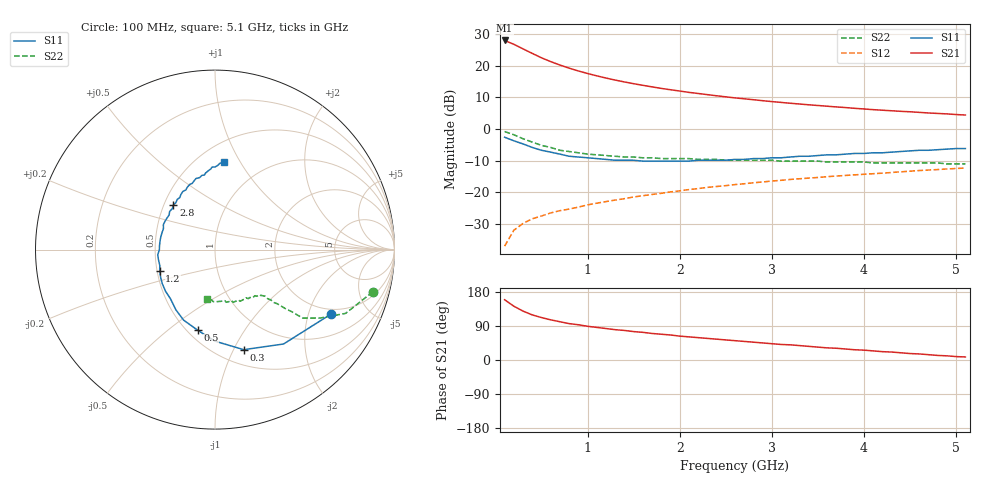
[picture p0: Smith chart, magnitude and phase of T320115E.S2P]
!AT-32011
!S PARAMETERS at Vce=5  V  Ic=10mA.  LAST UPDATED 01-05-95
# ghz s ma r 50
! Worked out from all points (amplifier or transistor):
!   51 points, 100 MHz to 5.1 GHz, reference 50 ohm
!   highest |S21| = 28.0 dB at 100 MHz (marker M1)
!   |S21| within 3 dB of that: start of sweep to 323.5 MHz
!   unconditionally stable (mu >= 1): 1.505 GHz to 4.873 GHz
!   at 900 MHz: K = 0.86, MSG = 21.5 dB, |S12| = -24.7 dB
!   at 2.6 GHz: K = 1.08, MAG = 11.9 dB, |S12| = -17.6 dB
!   at 5.1 GHz: K = 1.00, MSG = 8.4 dB, |S12| = -12.4 dB
!   S11 on the Smith chart (normalised r, x): 100 MHz: 1.79, -2.83; 300 MHz: 0.65, -1.10; 500 MHz: 0.56, -0.64; 1.2 GHz: 0.52, -0.14; 2.8 GHz: 0.56, +0.31; 5.1 GHz: 0.67, +0.86
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0.1  0.74 -29.0  25.11 159.0  0.014 76.0  0.91 -15.0
0.2  0.65 -54.0  21.83 142.0  0.025 66.0  0.81 -26.0
0.3  0.58 -74.0  18.48 129.0  0.032 60.0  0.7 -33.0
0.4  0.51 -90.0  15.67 119.0  0.038 57.0  0.62 -38.0
0.5  0.46 -102.0  13.35 112.0  0.042 56.0  0.55 -39.0
0.6  0.43 -114.0  11.62 106.0  0.047 55.0  0.51 -40.0
0.7  0.4 -123.0  10.26 101.0  0.051 55.0  0.46 -41.0
0.8  0.37 -132.0  9.16 96.0  0.054 55.0  0.44 -42.0
0.9  0.36 -140.0  8.27 93.0  0.058 55.0  0.42 -42.0
1  0.35 -147.0  7.54 89.0  0.063 56.0  0.4 -43.0
1.2  0.33 -159.0  6.39 83.0  0.071 56.0  0.38 -43.0
1.3  0.32 -164.0  5.93 80.0  0.075 56.0  0.37 -44.0
1.5  0.32 -175.0  5.2 75.0  0.084 56.0  0.36 -46.0
1.8  0.31 171.0  4.38 68.0  0.096 55.0  0.34 -49.0
2.1  0.31 158.0  3.79 61.0  0.11 54.0  0.34 -52.0
2.6  0.33 140.0  3.1 51.0  0.132 52.0  0.32 -59.0
2.8  0.34 133.0  2.9 47.0  0.141 50.0  0.32 -61.0
3.1  0.35 124.0  2.63 41.0  0.154 48.0  0.31 -65.0
3.5  0.38 114.0  2.35 34.0  0.171 46.0  0.31 -71.0
3.9  0.41 105.0  2.12 27.0  0.188 42.0  0.3 -76.0
4.3  0.43 97.0  1.94 21.0  0.205 40.0  0.29 -82.0
5.1  0.49 84.0  1.66 8.0  0.241 32.0  0.28 -99.0
